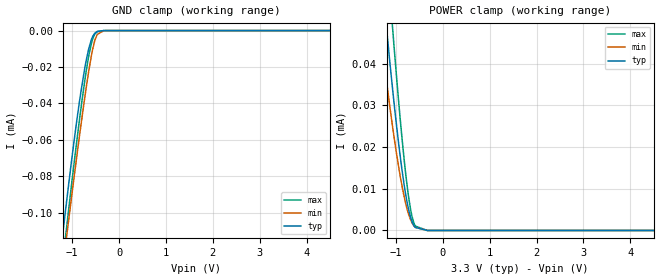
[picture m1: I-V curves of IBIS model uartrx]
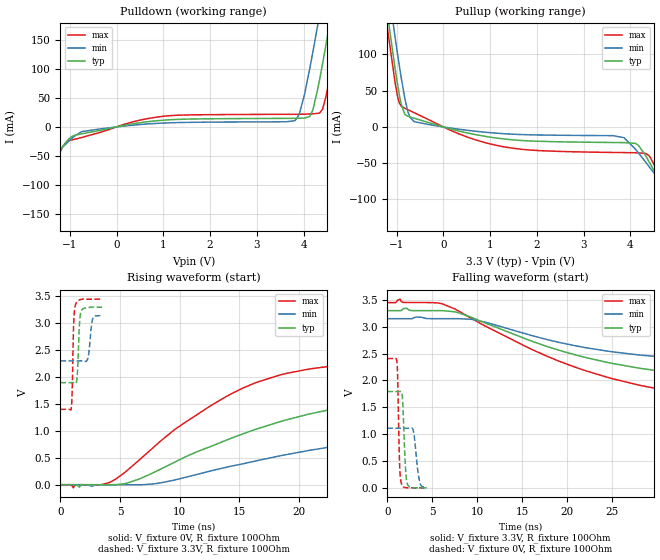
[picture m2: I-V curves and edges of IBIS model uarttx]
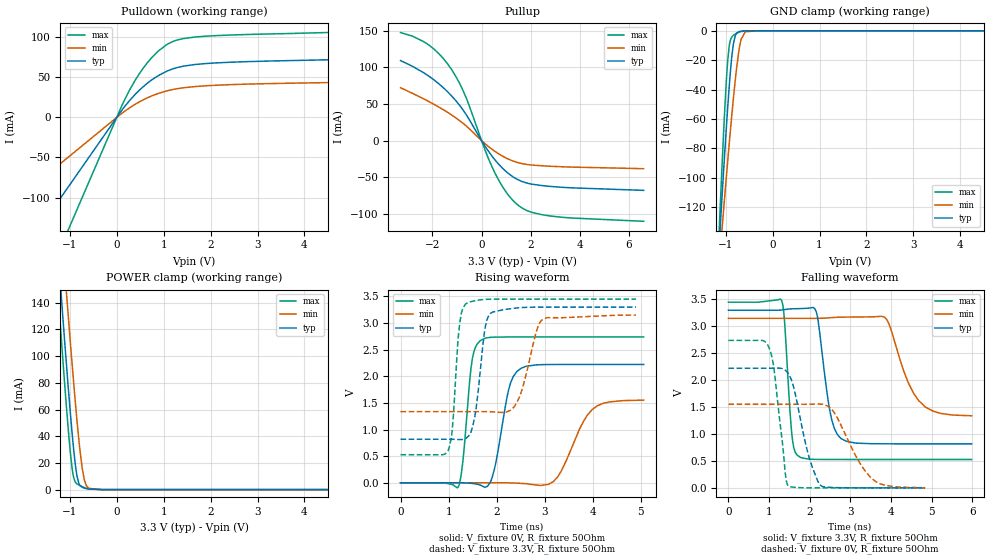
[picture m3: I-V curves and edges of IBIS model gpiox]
|Texas Instruments Incorporated
| Marketing part#   Digital Voltage Range   Package-type   #pins
| TPS65981   3.15V-3.45V   VQFN   56
[IBIS Ver]   4.1
[File name]   tps65981.ibs
[File Rev]   1.0
[Date]   8/3/2016
[Source]
| Texas Instruments Incorporated.
| Analog-eLab Design Center, HPA
| 12500 TI Blvd
| Dallas, TX -75243
[Notes]   Revision History:
| Rev 1.0: 8/3/2016
| - Initial version of the model
| - Model generated from simulations in TISPICE
| - Model matched to SPICE simulation
| - C_comp although listed in numerical order of value are
|   obtained from varying PVT conditions. For PVT conditions for
|   each specific value refer the buffer description under
|   respective [Model]. IBIS model user is responsible for using
|   appropriate C_comp to simulate for Signal Integrity.
[Disclaimer]
| This model is designed as an aid for customers of Texas Instruments.
| TI and its licensors and suppliers make no warranties, either expressed
| or implied, with respect to this  model, including the warranties of
| merchantability or fitness for a particular purpose. The model is
| provided solely on an "as is" basis. The entire risk as to its quality
| and performance is with the customer.
[Copyright]
(C) Copyright 2015 Texas Instruments Incorporated.All rights reserved.
|   TPS65982ZQZ
[Component]   TPS65981
[Manufacturer]   TI
[Package]   |56  -  VQFN package
|   typ   min   max
R_pkg   0.067   0.027   0.083
L_pkg   0.937nH   0.593nH   1.143nH
C_pkg   0.144pF   0.126pF   0.200pF
[Pin]  signal_name   model_name   R_pin   L_pin   C_pin
1   GPIO8   gpiols   NA   NA   NA
2   DEBUG1   gpiols   NA   NA   NA
3   SS   NC   NA   NA   NA
4   USB_RP_P   NC   NA   NA   NA
5   USB_RP_N   NC   NA   NA   NA
6   C_USB_TP   NC   NA   NA   NA
7   C_USB_TN   NC   NA   NA   NA
8   C_USB_BP   NC   NA   NA   NA
9   C_USB_BN   NC   NA   NA   NA
10   C_SBU1   NC   NA   NA   NA
11   C_SBU2   NC   NA   NA   NA
12   RPD_G1   NC   NA   NA   NA
13   C_CC1   NC   NA   NA   NA
14   PP_CABLE   POWER   NA   NA   NA
15   C_CC2   NC   NA   NA   NA
16   PD_G2   NC   NA   NA   NA
17   VBUS   POWER   NA   NA   NA
18   VBUS   POWER   NA   NA   NA
19   GPIO3   gpiols   NA   NA   NA
20   GPIO6   gpiols   NA   NA   NA
21   RESETZ   gpiols   NA   NA   NA
22   BUSPOWERZ   gpiols   NA   NA   NA
23   GPIO5   gpiols   NA   NA   NA
24   MRESET   gpiols   NA   NA   NA
25   GPIO2   gpiols   NA   NA   NA
26   GPIO4   gpiols   NA   NA   NA
27   PP_5V0   POWER   NA   NA   NA
28   PP_5V0   POWER   NA   NA   NA
29   SENSEN   NC   NA   NA   NA
30   SENSEP   NC   NA   NA   NA
31   HV_GATE1   NC   NA   NA   NA
32   HV_GATE2   NC   NA   NA   NA
33   PP_HV   POWER   NA   NA   NA
34   PP_HV   POWER   NA   NA   NA
35   SPI_MISO   gpiox   NA   NA   NA
36   SPI_MOSI   gpiox   NA   NA   NA
37   SPI_CLK   gpiox   NA   NA   NA
38   GPIO7   gpiols   NA   NA   NA
39   SPI_SSZ   gpiox   NA   NA   NA
40   LDO_1V8D   POWER   NA   NA   NA
41   GPIO0   gpiols   NA   NA   NA
42   VDDIO   POWER   NA   NA   NA
43   I2C_IRQZ   od   NA   NA   NA
44   DEBUG_CTL2   gpiols_i2c   NA   NA   NA
45   DEBUG_CTL1   gpiols_i2c   NA   NA   NA
46   I2C_SDA   sda   NA   NA   NA
47   I2C_SCL   scl   NA   NA   NA
48   LDO_BMC   POWER   NA   NA   NA
49   SWD_DATA   gpiox   NA   NA   NA
50   SWD_CLK   gpiox   NA   NA   NA
51   LDO_3V3   POWER   NA   NA   NA
52   R_OSC   NC   NA   NA   NA
53   VIN_3V3   POWER   NA   NA   NA
54   AUX_P   NC   NA   NA   NA
55   AUX_N   NC   NA   NA   NA
56   LDO_1V8A   POWER   NA   NA   NA
| Models and submodels in the file (8): uartrx (Input), uarttx (Output), gpiox (I/O), gpiols (I/O), gpiols_i2c (I/O), sda (I/O_open_drain), scl (I/O_open_drain), od (Open_sink)
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|   uartrx Model
[Model]   uartrx
Model_type   Input
Vinl = 0.80
Vinh = 2.00
|   typ   min   max
|   (nom PVT)   (fast PVT)   (slow PVT)
C_comp   1.884e-13   1.883e-13   1.922e-13
| Where nom  PVT is Nominal Process, 3.3V, 27C
|   Fast PVT is Strong Process,  3.45V, -40C
|   Slow PVT is Weak Process,   3.15V, 125C
[Voltage Range]   3.3   3.15   3.45
|Junction Temperature
[Temperature Range]   27   125   -40
[Power Clamp Reference]   3.3   3.15   3.45
[GND Clamp Reference]   0   0   0
[GND Clamp]
|   Voltage   I(typ)   I(min)   I(max)
-3.3V     -616.4uA   -586.9uA   -673.7uA
-1.268V   -126.8uA   -144.3uA   -142.4uA
-1.14V    -98.51uA   -117.6uA   -113uA
-1.033V   -75.66uA   -95.54uA   -89.02uA
-843.6mV  -38.94uA   -57.88uA   -48.92uA
-733.2mV  -21.02uA   -37.2uA    -27.92uA
-650.1mV  -10.41uA   -22.91uA   -14.51uA
-587.4mV  -4.818uA   -13.5uA    -6.861uA
-524.7mV  -1.682uA   -6.189uA   -2.313uA
-465mV    -476nA     -2.11uA    -584.1nA
-222.5mV  0A         0A         0A
6.6V      0A         0A         0A
[POWER Clamp]
|   Voltage   I(typ)   I(min)   I(max)
-3.3V     363.5uA    282.4uA    459.4uA
-1.331V   64.51uA    47.82uA    88.59uA
-1.206V   49.19uA    36.28uA    68.73uA
-1.122V   39.53uA    29.05uA    56.03uA
-1.061V   32.84uA    24.08uA    47.16uA
-906mV    17.59uA    12.89uA    26.45uA
-795.3mV  8.89uA     6.653uA    13.99uA
-729.8mV  5.015uA    3.913uA    8.085uA
-686.4mV  3.106uA    2.555uA    5.017uA
-588.3mV  737.6nA    762.5nA    1.066uA
-330mV    0A         11.44nA    0A
6.6V      0A         0A         0A
|   uarttx Model
[Model]   uarttx
Model_type   Output
Polarity   Non-Inverting
Vmeas = 1.65
Vref = 0
Cref = 2pF
Rref = 200
|   typ   min   max
|   (nom PVT)   (fast PVT)   (slow PVT)
C_comp   5.219e-13   4.960e-13   5.699e-13
| Where nom  PVT is Nominal Process, 3.3V, 27C
|   Fast PVT is Strong Process,  3.45V, -40C
|   Slow PVT is Weak Process,   3.15V, 125C
[Voltage Range]   3.3   3.15   3.45
|Junction Temperature
[Temperature Range]   27   125   -40
[Pullup Reference]   3.3   3.15   3.45
[Pulldown Reference]   0   0   0
[Power Clamp Reference]   3.3   3.15   3.45
[GND Clamp Reference]   0   0   0
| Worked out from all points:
|   slope of the pulldown table from 0 to 0.495 V, typ, clamps not added: 68.4 ohm
|   slope of the pullup table from 0 to 0.495 V, typ, clamps not added: 61.3 ohm
|   falling waveform, V_fixture 3.3V, R_fixture 100Ohm: 20-80 % time 18.5ns typ, 15.1ns min, 20.5ns max; typ from 3.3 V to 1.9 V
|   rising waveform, V_fixture 0V, R_fixture 100Ohm: 20-80 % time 14.5ns typ, 17.7ns min, 10.1ns max; typ from 0 V to 1.79 V
|   rising waveform, V_fixture 3.3V, R_fixture 100Ohm: 20-80 % time 158ps typ, 228ps min, 128ps max; typ from 1.9 V to 3.3 V
|   falling waveform, V_fixture 0V, R_fixture 100Ohm: 20-80 % time 271ps typ, 426ps min, 190ps max; typ from 1.79 V to 0.001 V
[Pulldown]
|   Voltage   I(typ)   I(min)   I(max)
-3.3V     -295.9mA   -222.5mA   -395.2mA
-1.723V   -100.8mA   -83.38mA   -125.5mA
-1.155V   -34.06mA   -35.23mA   -34.78mA
-742.2mV  -11.87mA   -8.083mA   -18.25mA
1.053V    11.95mA    6.868mA    18.86mA
3.819V    14.88mA    10.9mA     21.89mA
4.134V    18.24mA    101.1mA    22.45mA
4.31V     67.66mA    179mA      23.58mA
4.559V    178.9mA    295.7mA    85.55mA
4.683V    237.9mA    355.2mA    142.3mA
5.019V    401.4mA    518.3mA    305.3mA
6.6V      1.193A     1.302A     1.105A
[Pullup]
|   Voltage   I(typ)   I(min)   I(max)
-3.3V     1.215A     1.243A     1.21A
-1.216V   164.2mA    207.6mA    144.4mA
-1.037V   81.83mA    125.1mA    62.46mA
-943.8mV  44.61mA    84.81mA    33.37mA
-761.1mV  14.82mA    21.36mA    23.8mA
-625.7mV  12.02mA    7.365mA    19.69mA
1.251V    -16.27mA   -9.155mA   -26.91mA
3.866V    -21.63mA   -14.87mA   -35.39mA
4.156V    -24.62mA   -34.6mA    -35.75mA
4.411V    -49.17mA   -55.61mA   -40.34mA
5.087V    -130.2mA   -114.2mA   -146.2mA
6.6V      -317.9mA   -248.2mA   -405.3mA
[Ramp]
R_load = 100
|   typ   min   max
dV/dt_r   1.07582/1.45421e-08   0.66599/1.79204e-08   1.44461/1.00345e-08
dV/dt_f   0.841274/1.8421e-08   0.509094/1.51105e-08   1.22678/2.04399e-08
[Falling Waveform]
V_fixture = 3.3V
V_fixture_min = 3.15V
V_fixture_max = 3.45V
R_fixture = 100Ohm
|   Time   V(typ)   V(min)   V(max)
0s        3.3V       3.15V      3.45V
1.422ns   3.3V       3.15V      3.514V
1.766ns   3.336V     3.15V      3.453V
6.178ns   3.3V       3.151V     3.423V
10.67ns   3.084V     3.093V     3.032V
21.09ns   2.469V     2.64V      2.236V
27.88ns   2.233V     2.477V     1.918V
35.79ns   2.076V     2.382V     1.696V
57.46ns   1.929V     2.311V     1.47V
100ns     1.898V     2.302V     1.405V
[Rising Waveform]
V_fixture = 0V
V_fixture_min = 0V
V_fixture_max = 0V
R_fixture = 100Ohm
|   Time   V(typ)   V(min)   V(max)
0s        1.779nV    51.61nV    941pV
1.08ns    39.41uV    50.68nV    -58.51mV
4.122ns   -2.492mV   -38.34uV   41.13mV
8.372ns   285.5mV    32.82mV    804.4mV
14.01ns   834.7mV    329.1mV    1.649V
16.42ns   1.031V     442.7mV    1.898V
21.06ns   1.322V     643.8mV    2.155V
26.85ns   1.542V     821.9mV    2.282V
36.28ns   1.694V     980.9mV    2.36V
71.83ns   1.789V     1.104V     2.406V
[Rising Waveform]
V_fixture = 3.3V
V_fixture_min = 3.15V
V_fixture_max = 3.45V
R_fixture = 100Ohm
|   Time   V(typ)   V(min)   V(max)
0s        1.897V     2.301V     1.401V
900ps     1.897V     2.301V     1.406V
974ps     1.897V     2.301V     1.674V
1.128ns   1.896V     2.301V     3.084V
1.292ns   1.884V     2.301V     3.362V
1.416ns   2.041V     2.301V     3.405V
1.738ns   3.227V     2.302V     3.443V
2.308ns   3.293V     2.349V     3.446V
2.712ns   3.3V       3.083V     3.447V
3.486ns   3.297V     3.146V     3.447V
[Falling Waveform]
V_fixture = 0V
V_fixture_min = 0V
V_fixture_max = 0V
R_fixture = 100Ohm
|   Time   V(typ)   V(min)   V(max)
0s        1.794V     1.111V     2.408V
1.054ns   1.794V     1.111V     2.368V
1.148ns   1.794V     1.111V     2.067V
1.366ns   1.793V     1.111V     441.7mV
1.564ns   1.79V      1.111V     80.61mV
1.696ns   1.639V     1.111V     31.2mV
2.19ns    90.75mV    1.111V     2.688mV
2.864ns   3.776mV    1.084V     739.1uV
3.594ns   1.059mV    113.8mV    742uV
4.408ns   691.5uV    4.016mV    764uV
|   gpiox Model
[Model]   gpiox
Model_type   I/O
Polarity   Non-Inverting
Enable   Active-High
Vinl = 0.80
Vinh = 2.00
Vmeas = 1.65
Vref = 0
Cref = 2pF
Rref = 100
|   typ   min   max
|   (nom PVT)   (fast PVT)   (slow PVT)
C_comp   1.059e-12   1.036e-12   1.086e-12
| Where nom  PVT is Nominal Process, 3.3V, 27C
|   Fast PVT is Strong Process,  3.45V, -40C
|   Slow PVT is Weak Process,   3.15V, 125C
[Voltage Range]   3.3   3.15   3.45
|Junction Temperature
[Temperature Range]   27   125   -40
[Pullup Reference]   3.3   3.15   3.45
[Pulldown Reference]   0   0   0
[Power Clamp Reference]   3.3   3.15   3.45
[GND Clamp Reference]   0   0   0
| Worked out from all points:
|   slope of the pulldown table from 0 to 0.495 V, typ, clamps not added: 14.3 ohm
|   slope of the pullup table from 0 to 0.495 V, typ, clamps not added: 20.4 ohm
|   GND clamp passes 1 mA (typ) near -0.74 V on its own axis
|   POWER clamp passes 1 mA (typ) near -0.68 V on its own axis
|   falling waveform, V_fixture 3.3V, R_fixture 50Ohm: 20-80 % time 269ps typ, 546ps min, 145ps max; typ from 3.3 V to 0.818 V
|   rising waveform, V_fixture 0V, R_fixture 50Ohm: 20-80 % time 262ps typ, 477ps min, 159ps max; typ from 0 V to 2.22 V
|   rising waveform, V_fixture 3.3V, R_fixture 50Ohm: 20-80 % time 184ps typ, 301ps min, 129ps max; typ from 0.818 V to 3.3 V
|   falling waveform, V_fixture 0V, R_fixture 50Ohm: 20-80 % time 402ps typ, 647ps min, 241ps max; typ from 2.22 V to 0 V
[Pulldown]
|   Voltage   I(typ)   I(min)   I(max)
-3.3V     -277mA     -158.5mA   -447.7mA
-150.2mV  -12.61mA   -7.21mA    -20.37mA
151.8mV   12.28mA    6.938mA    20.02mA
274.2mV   21.1mA     11.96mA    34.21mA
460.5mV   32.75mA    18.65mA    52.7mA
653.4mV   42.71mA    24.42mA    68.26mA
854.7mV   51.01mA    29.25mA    81.01mA
1.178V    60.18mA    34.6mA     94.27mA
1.422V    63.9mA     36.96mA    98.32mA
2.041V    67.72mA    39.9mA     101.8mA
5.432V    73.05mA    44.32mA    107.3mA
6.6V      76.33mA    46.37mA    112.1mA
[GND Clamp]
|   Voltage   I(typ)   I(min)   I(max)
-3.3V     -1.417A    -1.066A    -1.893A
-1.199V   -179.2mA   -182.9mA   -181.3mA
-1.116V   -133.7mA   -150mA     -119.5mA
-1.076V   -112.1mA   -134.2mA   -90.78mA
-988.5mV  -67.46mA   -100.7mA   -35.54mA
-953.7mV  -50.94mA   -87.68mA   -19.31mA
-909.2mV  -31.72mA   -71.45mA   -7.69mA
-838.2mV  -9.42mA    -46.98mA   -3.178mA
-720.1mV  -595uA     -13.97mA   -982.8uA
-581.6mV  -40.13uA   -626.1uA   -81.68uA
-330mV    -70.13nA   -605.5nA   -45.49nA
6.6V      0A         0A         0A
[Pullup]
|   Voltage   I(typ)   I(min)   I(max)
-3.3V     109.3mA    72.2mA     147.5mA
-2.134V   87.66mA    53.06mA    130.1mA
-1.567V   72.53mA    42.38mA    112.5mA
-1.216V   60.85mA    34.92mA    96.78mA
-626.2mV  35.49mA    20.06mA    58.32mA
146.6mV   -7.842mA   -4.352mA   -13.36mA
521.4mV   -25.32mA   -14.14mA   -42.61mA
1.053V    -43.8mA    -24.62mA   -72.71mA
1.475V    -53.28mA   -29.99mA   -87.89mA
2.005V    -59.17mA   -33.21mA   -97.51mA
2.831V    -62.63mA   -35.06mA   -103.1mA
6.6V      -67.93mA   -38.33mA   -110.2mA
[POWER Clamp]
|   Voltage   I(typ)   I(min)   I(max)
-3.3V     1.237A     1.263A     1.239A
-1.258V   181mA      234.5mA    150.2mA
-1.144V   126.7mA    180.8mA    94.91mA
-1.076V   95.5mA     149.5mA    63.67mA
-1.033V   76.43mA    130.1mA    45.13mA
-990mV    57.86mA    110.8mA    28.14mA
-930.6mV  34.46mA    85.16mA    11.11mA
-844.8mV  9.689mA    50.62mA    4.235mA
-739mV    1.755mA    16.64mA    2.217mA
-647mV    743.2uA    2.889mA    1.001mA
-330mV    1.406uA    4.138uA    685.6nA
6.6V      0A         0A         0A
[Ramp]
R_load = 50
|   typ   min   max
dV/dt_r   1.33389/2.60015e-10   0.931714/4.70432e-10   1.64372/1.58172e-10
dV/dt_f   1.48927/2.68363e-10   1.08801/5.43452e-10   1.75377/1.45042e-10
[Falling Waveform]
V_fixture = 3.3V
V_fixture_min = 3.15V
V_fixture_max = 3.45V
R_fixture = 50Ohm
|   Time   V(typ)   V(min)   V(max)
0s        3.3V       3.15V      3.45V
1.306ns   3.305V     3.15V      3.488V
1.56ns    3.326V     3.15V      997mV
1.7ns     3.329V     3.15V      600.9mV
2.16ns    3.271V     3.149V     528.9mV
2.51ns    1.375V     3.162V     527.5mV
2.776ns   913.8mV    3.172V     527.2mV
3.83ns    818.6mV    3.175V     527.1mV
4.68ns    817.9mV    1.622V     527.1mV
5.982ns   817.9mV    1.339V     527.1mV
[Rising Waveform]
V_fixture = 0V
V_fixture_min = 0V
V_fixture_max = 0V
R_fixture = 50Ohm
|   Time   V(typ)   V(min)   V(max)
0s        505.5pV    14.97nV    196.3pV
1.202ns   574.3uV    426.7nV    -79.46mV
1.494ns   -12.58mV   -3.585uV   2.327V
1.654ns   -41.27mV   -26.69uV   2.667V
1.886ns   49.79mV    228.1uV    2.733V
2.242ns   1.722V     -1.633mV   2.739V
2.508ns   2.151V     -11.3mV    2.739V
3.186ns   2.222V     27.84mV    2.74V
4.09ns    2.223V     1.444V     2.74V
5.058ns   2.223V     1.553V     2.74V
[Rising Waveform]
V_fixture = 3.3V
V_fixture_min = 3.15V
V_fixture_max = 3.45V
R_fixture = 50Ohm
|   Time   V(typ)   V(min)   V(max)
0s        817.9mV    1.337V     527mV
988ps     818.1mV    1.337V     597.7mV
1.078ns   817.6mV    1.337V     1.024V
1.236ns   811.5mV    1.337V     3.021V
1.36ns    832.2mV    1.337V     3.362V
1.55ns    1.265V     1.337V     3.419V
1.874ns   3.184V     1.335V     3.448V
2.426ns   3.285V     1.52V      3.45V
2.932ns   3.3V       3.052V     3.45V
4.898ns   3.3V       3.15V      3.45V
[Falling Waveform]
V_fixture = 0V
V_fixture_min = 0V
V_fixture_max = 0V
R_fixture = 50Ohm
|   Time   V(typ)   V(min)   V(max)
0s        2.223V     1.553V     2.74V
1.002ns   2.223V     1.553V     2.599V
1.104ns   2.224V     1.553V     2.299V
1.394ns   2.189V     1.553V     301.3mV
1.472ns   2.124V     1.553V     36.68mV
2.002ns   520.6mV    1.554V     770.1uV
2.25ns    57.55mV    1.557V     204.5uV
2.606ns   6.093mV    1.393V     39.09uV
3.616ns   37.19uV    119.7mV    1.922uV
4.838ns   1.764uV    1.853mV    717.1nV
